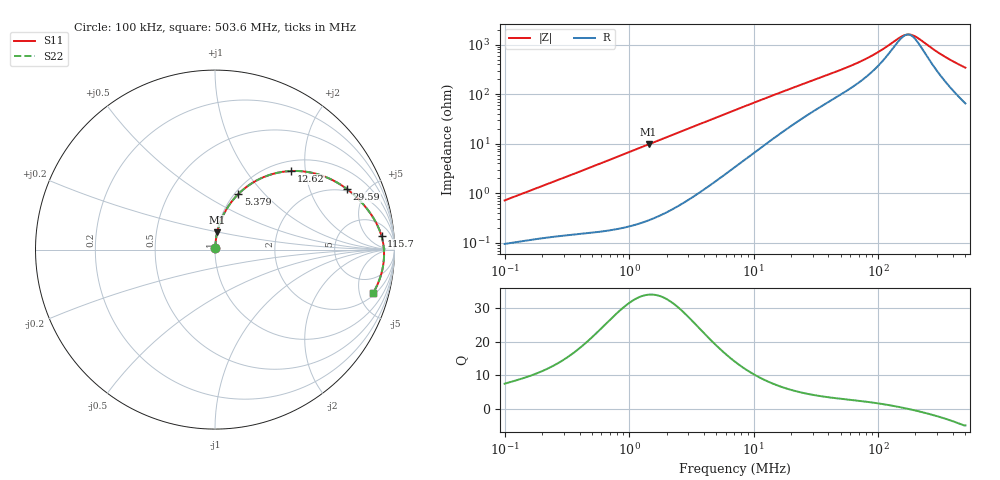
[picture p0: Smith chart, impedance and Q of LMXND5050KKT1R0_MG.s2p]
! LMXND5050KKT1R0_MG  S-PARAMETER MODEL  ( General Type )
! Model Generated by TAIYO YUDEN Corporation (http://www.ty-top.com)
! Version 1.0
! TAIYO YUDEN Control No. 191023NI43SB-FBB
! Copyright(c) 2019 TAIYO YUDEN CO.,LTD. All Rights Reserved.
! Product Description (link to TY-COMPAS)
! https://ds.yuden.co.jp/TYCOMPAS/or/detail?pn=LMXND5050KKT1R0NMG&u=M
! Products Name : Inductors
! Characteristics :
!  Inductance : 1.0 uH , SRF(min) : 95 MHz , DC Resistance(max) : 0.084 Ohm
!  Rated Current : Saturation :2350 mA , Temp Rise : 1750 mA
!  Case Size : 4.9 x 4.9 / 0.193 x 0.193 [mm/inch] , Thickness : 1 / 0.039 [mm/inch]
!  (Conditions: Temperature = 25 degC , DC Bias Current/Voltage = 0A / 0V)
! External Node Assignments :
!  1  o---GGG---o  2
! GND o---------o GND
! Frequency Range : 0.1MHz  -  503.601575MHz  [ 402 STEP ]
# MHz S RI R 50
! Freq[MHz].  S11 Real  S11 Imag  S21 Real  S21 Imag  S12 Real  S12 Imag  S22 Real  S22 Imag
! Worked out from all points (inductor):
!   401 points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, 100 kHz to 503.6 MHz, reference 50 ohm
!   read as one part in series: L = 1.12 uH near 104.4 kHz
!   highest Q = 34.1 at 1.435 MHz (marker M1), where L = 1.08 uH
!   self-resonance near 172.4 MHz
!   S11 on the Smith chart (normalised r, x): 100 kHz: 1.00, +0.01; 5.379 MHz: 1.04, +0.72; 12.62 MHz: 1.20, +1.67; 29.59 MHz: 1.87, +3.65; 115.7 MHz: 12, +14; 503.6 MHz: 2.30, -6.72
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0.1  0.001 0.00711  0.999 -0.00711  0.999 -0.00711  0.001 0.00711
0.416965  0.00233 0.0283  0.9977 -0.0283  0.9977 -0.0283  0.00233 0.0283
1.435166  0.0121 0.0956  0.9879 -0.0956  0.9879 -0.0956  0.0121 0.0956
1.738598  0.0169 0.1151  0.9831 -0.1151  0.9831 -0.1151  0.0169 0.1151
3.295002  0.0544 0.2084  0.9456 -0.2084  0.9456 -0.2084  0.0544 0.2084
5.379299  0.1293 0.3088  0.8707 -0.3088  0.8707 -0.3088  0.1293 0.3088
7.249345  0.2084 0.3715  0.7916 -0.3715  0.7916 -0.3715  0.2084 0.3715
9.769488  0.3152 0.4196  0.6848 -0.4196  0.6848 -0.4196  0.3152 0.4196
12.61637  0.422 0.4378  0.578 -0.4378  0.578 -0.4378  0.422 0.4378
18.1248  0.5734 0.4195  0.4266 -0.4195  0.4266 -0.4195  0.5734 0.4195
29.58987  0.7338 0.3383  0.2662 -0.3383  0.2662 -0.3383  0.7338 0.3383
43.42472  0.8172 0.2623  0.1828 -0.2623  0.1828 -0.2623  0.8172 0.2623
66.50302  0.8801 0.1802  0.1199 -0.1802  0.1199 -0.1802  0.8801 0.1802
89.62196  0.9102 0.1239  0.0898 -0.1239  0.0898 -0.1239  0.9102 0.1239
115.7383  0.9278 0.0758  0.0722 -0.0758  0.0722 -0.0758  0.9278 0.0758
123.3794  0.931 0.0638  0.069 -0.0638  0.069 -0.0638  0.931 0.0638
159.3329  0.9398 0.0152  0.0602 -0.0152  0.0602 -0.0152  0.9398 0.0152
173.5107  0.9412 -0.0012  0.0588 0.0012  0.0588 0.0012  0.9412 -0.0012
184.966  0.9418 -0.0136  0.0582 0.0136  0.0582 0.0136  0.9418 -0.0136
210.1954  0.9418 -0.0389  0.0582 0.0389  0.0582 0.0389  0.9418 -0.0389
343.1572  0.9239 -0.1443  0.0761 0.1443  0.0761 0.1443  0.9239 -0.1443
503.6016  0.8823 -0.2398  0.1177 0.2398  0.1177 0.2398  0.8823 -0.2398
